(* Logix 5000 AddOnInstructionDefinition export RTA_SCNDR_P1_Barcode_Scanner_to_PLC_AOI; software revision 32.00 *)

TYPE RTA_STRING_4096 :   // string type; String data type with up to 4096 characters available.
STRUCT
   LEN : DINT;
   DATA : SINT[4096];
END_STRUCT
END_TYPE

ADD_ON_INSTRUCTION RTA_SCNDR_P1_Barcode_Scanner_to_PLC_AOI   (* revision 1.0, vendor Real Time Automation, Inc. *)
// RTA's 435NBX gateway to PLC handshaking
VAR_IN_OUT
   DataIn : RTA_STRING_4096; {required}
   DataOut : RTA_STRING_4096; {required}
   GarbageData : BOOL; {required}   // The Barcode Scanner is unplugged / unpowered
END_VAR
VAR
   CR_Offset : DINT; {access None}
   LF_Offset : DINT; {access None}
   LF : RTA_STRING_4096 := '$l'; {access None}
   CR : RTA_STRING_4096 := '$r'; {access None}
END_VAR

ROUTINE Logic   (* ladder *)
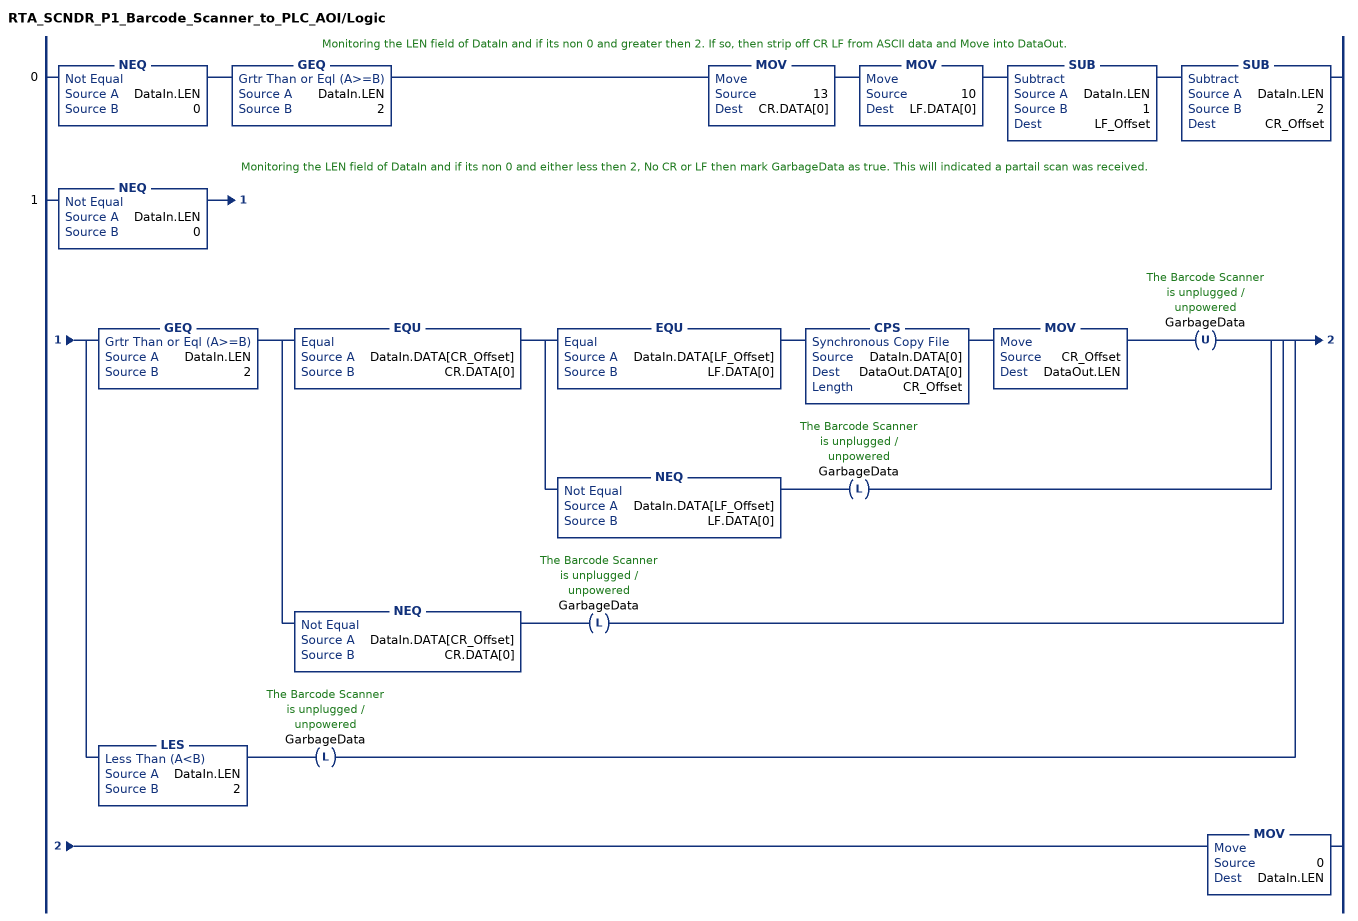
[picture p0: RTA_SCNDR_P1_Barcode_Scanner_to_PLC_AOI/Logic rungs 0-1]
   // Monitoring the LEN field of DataIn and if its non 0 and greater then 2. If so, then strip off CR LF from ASCII data and Move into DataOut.
   0: NEQ(DataIn.LEN,0)GEQ(DataIn.LEN,2)MOV(13,CR.DATA[0])MOV(10,LF.DATA[0])SUB(DataIn.LEN,1,LF_Offset)SUB(DataIn.LEN,2,CR_Offset);
   // Monitoring the LEN field of DataIn and if its non 0 and either less then 2, No CR or LF then mark GarbageData as true. This will indicated a partail scan was received.
   1: NEQ(DataIn.LEN,0)[GEQ(DataIn.LEN,2) [EQU(DataIn.DATA[CR_Offset],CR.DATA[0]) [EQU(DataIn.DATA[LF_Offset],LF.DATA[0]) CPS(DataIn.DATA[0],DataOut.DATA[0],CR_Offset) MOV(CR_Offset,DataOut.LEN) OTU(GarbageData) ,NEQ(DataIn.DATA[LF_Offset],LF.DATA[0]) OTL(GarbageData) ] ,NEQ(DataIn.DATA[CR_Offset],CR.DATA[0]) OTL(GarbageData) ] ,LES(DataIn.LEN,2) OTL(GarbageData) ]MOV(0,DataIn.LEN);
END_ROUTINE
END_ADD_ON_INSTRUCTION
